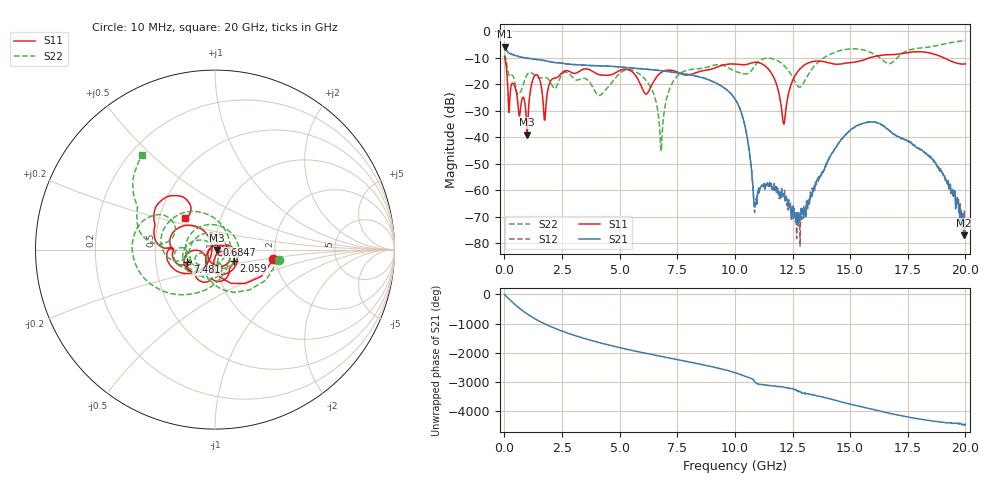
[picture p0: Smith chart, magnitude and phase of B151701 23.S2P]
!  2-Port S-parameters saved by WinCal
! VAR MeasName=S-Parameters (CALIBRATED_DATA) read from VNA (N5244A)
! VAR MeasDate=2015-12-24 19:10:50
! VAR NAME=B151701 23
! VAR FILENAME=B151701 23.S2P
! VAR DATE=2015-12-24 19:10:50
! VAR PHYS_PORTS=1,3
# Hz S DB R 50
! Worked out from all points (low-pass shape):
!   801 points, 10 MHz to 20 GHz, reference 50 ohm
!   highest |S21| = -5.92 dB at 10 MHz (marker M1); lowest = -77.0 dB at 19.93 GHz (marker M2)
!   |S21| within 3 dB of the highest: start of sweep to 363.2 MHz
!   lowest |S11| = -39.0 dB at 984.5 MHz (marker M3), VSWR 1.02, Z = 51 - j0.454 ohm
!   |S11| at or under -10 dB: 20.45 MHz to 15.9 GHz (15.87 GHz wide, 199 % of centre); 19.04 GHz to end of sweep
!   |S22| runs from -45.3 to -3.6 dB; largest |S21 - S12| = 0.0011
!   S11 on the Smith chart (normalised r, x): 10 MHz: 1.95, -0.23; 684.7 MHz: 1.02, +0.06; 2.059 GHz: 1.22, -0.16; 7.481 GHz: 0.73, -0.10; 20 GHz: 0.68, +0.25
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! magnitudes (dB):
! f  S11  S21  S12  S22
! 10 MHz  -9.6  -5.9  -5.9  -8.9
! 684.7 MHz  -30.4  -9.8  -9.8  -23.1
! 984.5 MHz  -39.0  -10.2  -10.2  -16.4
! 1.309 GHz  -16.9  -10.7  -10.6  -16.6
! 1.759 GHz  -33.6  -11.1  -11.1  -17.5
! 2.059 GHz  -18.2  -11.7  -11.7  -20.3
! 3.358 GHz  -14.6  -12.8  -12.8  -17.9
! 5.707 GHz  -16.9  -14.1  -14.1  -15.4
! 6.682 GHz  -16.5  -14.8  -14.8  -31.8
! 6.832 GHz  -15.4  -15.0  -15.0  -40.8
! 7.481 GHz  -15.4  -15.7  -15.7  -17.1
! 10.01 GHz  -12.4  -25.6  -25.6  -15.2
! 10.45 GHz  -12.7  -36.5  -36.5  -16.2
! 10.9 GHz  -11.8  -65.3  -63.4  -12.7
! 12.13 GHz  -35.1  -62.3  -60.9  -13.0
! 12.73 GHz  -15.3  -69.8  -71.4  -20.7
! 13.35 GHz  -11.6  -62.2  -59.1  -14.2
! 15.05 GHz  -11.9  -37.1  -37.1  -6.7
! 16.68 GHz  -8.9  -37.5  -37.2  -12.3
! 18.65 GHz  -8.8  -49.1  -49.5  -5.7
! 19.93 GHz  -12.5  -77.0  -71.7  -3.6
! 20 GHz  -12.4  -73.0  -71.0  -3.6
